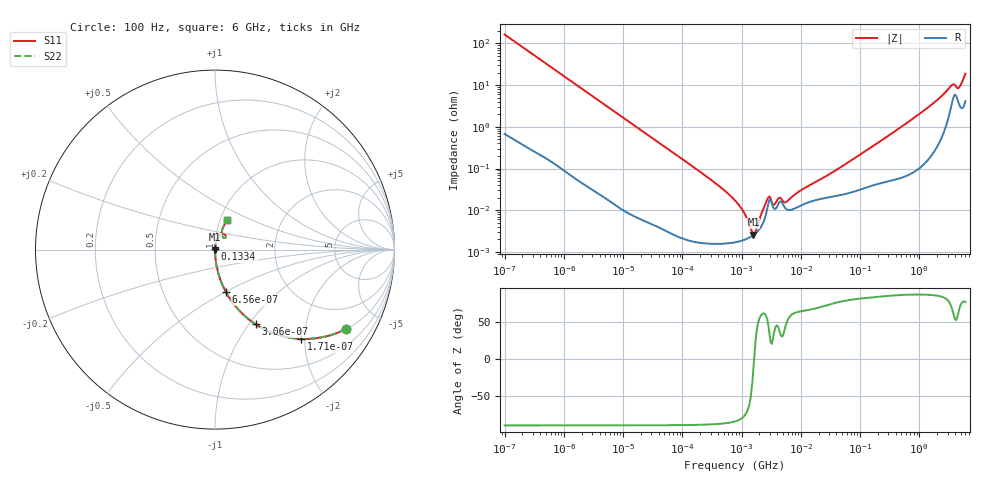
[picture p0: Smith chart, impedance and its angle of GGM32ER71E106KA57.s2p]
!Murata Part Number: GGM32ER71E106KA57
!These Parameters are Measured in Series Mode Connection
!Data Generated on Jun 19, 2026
!  o--ll--o
!Port1  Port2
!  o------o
!Operation Temp=25[degC], DC Bias Voltage=0[V]
!Freq. Start=100[Hz] Stop=6[GHz] 401[Steps]
# Hz S RI R 50
!Freq.(Hz) S11(Real) S11(Imag) S21(Real) S21(Imag) S12(Real) S12(Imag) S22(Real) S22(Imag)
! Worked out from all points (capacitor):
!   401 points, 100 Hz to 6 GHz, reference 50 ohm
!   read as one part in series: C = 9.67 uF near 109 Hz
!   lowest |Z| = 2.6 mohm at 1.586 MHz (marker M1)
!   series resonance near 1.625 MHz, so ESL is about 990 pH
!   S11 on the Smith chart (normalised r, x): 100 Hz: 1.01, -3.29; 171 Hz: 1.01, -1.92; 306 Hz: 1.01, -1.08; 656 Hz: 1.00, -0.50; 133.4 MHz: 1.00, +0.01; 6 GHz: 1.08, +0.37
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100  0.7289 -0.4425  0.2711 0.4425  0.2711 0.4425  0.7289 -0.4425
171  0.4804 -0.4974  0.5196 0.4974  0.5196 0.4974  0.4804 -0.4974
306  0.2256 -0.4156  0.7744 0.4156  0.7744 0.4156  0.2256 -0.4156
656  0.0609 -0.2364  0.9391 0.2364  0.9391 0.2364  0.0609 -0.2364
2008  0.00722 -0.082  0.9928 0.082  0.9928 0.082  0.00722 -0.082
40335  5.56e-05 -0.00415  0.9999 0.00415  0.9999 0.00415  5.56e-05 -0.00415
330837  1.58e-05 -0.000489  1 0.000489  1 0.000489  1.58e-05 -0.000489
774597  1.69e-05 -0.00017  1 0.00017  1 0.00017  1.69e-05 -0.00017
1059725  1.9e-05 -9.39e-05  1 9.39e-05  1 9.39e-05  1.9e-05 -9.39e-05
1585629  2.54e-05 -5.4e-06  1 5.4e-06  1 5.4e-06  2.54e-05 -5.4e-06
2169299  4.16e-05 7.19e-05  1 -7.19e-05  1 -7.19e-05  4.16e-05 7.19e-05
2837864  0.000145 0.000146  0.9999 -0.000146  0.9999 -0.000146  0.000145 0.000146
3549919  0.000108 8.02e-05  0.9999 -8.02e-05  0.9999 -8.02e-05  0.000108 8.02e-05
4440638  0.000162 0.000117  0.9998 -0.000117  0.9998 -0.000117  0.000162 0.000117
5809218  0.000104 0.000123  0.9999 -0.000123  0.9999 -0.000123  0.000104 0.000123
1.555665e7  0.000165 0.000395  0.9998 -0.000395  0.9998 -0.000395  0.000165 0.000395
1.334425e8  0.000365 0.0028  0.9996 -0.0028  0.9996 -0.0028  0.000365 0.0028
3.124326e8  0.000539 0.00631  0.9995 -0.00631  0.9995 -0.00631  0.000539 0.00631
1.497423e9  0.00277 0.0311  0.9972 -0.0311  0.9972 -0.0311  0.00277 0.0311
3.505958e9  0.0405 0.0863  0.9595 -0.0863  0.9595 -0.0863  0.0405 0.0863
4.586474e9  0.0419 0.07  0.9581 -0.07  0.9581 -0.07  0.0419 0.07
6e9  0.0684 0.164  0.9316 -0.164  0.9316 -0.164  0.0684 0.164
